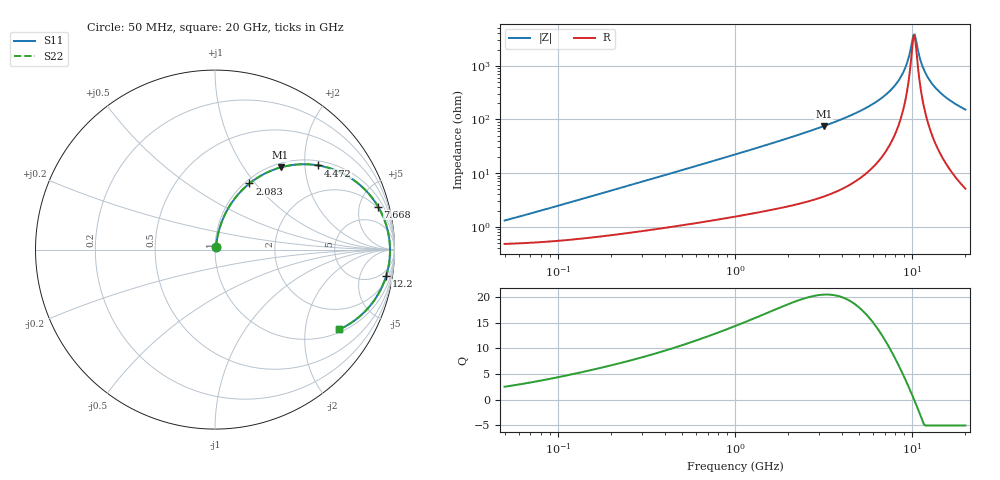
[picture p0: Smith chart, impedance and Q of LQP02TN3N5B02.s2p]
!Murata Part Number: LQP02TN3N5B02
!These Parameters are Measured in Series Mode Connection
!  o--[Z]--o
!Port1  Port2
!  o-------o
!Freq. Start=50[MHz] Stop=20[GHz], 401[Steps]
# Hz S RI R 50
!Freq.(Hz) S11(Real) S11(Imag) S21(Real) S21(Imag) S12(Real) S12(Imag) S22(Real) S22(Imag)
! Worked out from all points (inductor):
!   401 points, 50 MHz to 20 GHz, reference 50 ohm
!   read as one part in series: L = 3.85 nH near 61.67 MHz
!   highest Q = 20.5 at 3.169 GHz (marker M1), where L = 3.76 nH
!   self-resonance near 10.19 GHz
!   S11 on the Smith chart (normalised r, x): 50 MHz: 1.01, +0.02; 2.083 GHz: 1.05, +0.93; 4.472 GHz: 1.12, +2.35; 7.668 GHz: 1.78, +7.28; 12.2 GHz: 3, -12; 20 GHz: 1.10, -3.04
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5e7  0.00492 0.0121  0.9951 -0.0121  0.9951 -0.0121  0.00492 0.0121
1.364002e8  0.00702 0.032  0.993 -0.032  0.993 -0.032  0.00702 0.032
3.721004e8  0.0161 0.0826  0.9839 -0.0826  0.9839 -0.0826  0.0161 0.0826
1e9  0.0599 0.205  0.9401 -0.205  0.9401 -0.205  0.0599 0.205
2.083303e9  0.1921 0.3683  0.8079 -0.3683  0.8079 -0.3683  0.1921 0.3683
2.728004e9  0.2927 0.4309  0.7073 -0.4309  0.7073 -0.4309  0.2927 0.4309
3.168813e9  0.3655 0.4578  0.6345 -0.4578  0.6345 -0.4578  0.3655 0.4578
4.472136e9  0.5761 0.4688  0.4239 -0.4688  0.4239 -0.4688  0.5761 0.4688
5.944466e9  0.7684 0.3904  0.2316 -0.3904  0.2316 -0.3904  0.7684 0.3904
7.442007e9  0.8952 0.261  0.1048 -0.261  0.1048 -0.261  0.8952 0.261
7.668323e9  0.9085 0.2397  0.0915 -0.2397  0.0915 -0.2397  0.9085 0.2397
8.389408e9  0.9419 0.1712  0.0581 -0.1712  0.0581 -0.1712  0.9419 0.1712
9.041845e9  0.9614 0.1098  0.0386 -0.1098  0.0386 -0.1098  0.9614 0.1098
9.457416e9  0.9691 0.0717  0.0309 -0.0717  0.0309 -0.0717  0.9691 0.0717
1.004137e10  0.9746 0.0199  0.0254 -0.0199  0.0254 -0.0199  0.9746 0.0199
1.019291e10  0.9751 0.00689  0.0249 -0.00689  0.0249 -0.00689  0.9751 0.00689
1.050288e10  0.975 -0.0192  0.025 0.0192  0.025 0.0192  0.975 -0.0192
1.131968e10  0.9686 -0.0841  0.0314 0.0841  0.0314 0.0841  0.9686 -0.0841
1.220001e10  0.9537 -0.1473  0.0463 0.1473  0.0463 0.1473  0.9537 -0.1473
1.334722e10  0.925 -0.2192  0.075 0.2192  0.075 0.2192  0.925 -0.2192
1.482269e10  0.8785 -0.2949  0.1215 0.2949  0.1215 0.2949  0.8785 -0.2949
2e10  0.6926 -0.4449  0.3074 0.4449  0.3074 0.4449  0.6926 -0.4449
